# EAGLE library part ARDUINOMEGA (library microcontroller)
The Arduino Mega is a microcontroller board based on the ATmega1280. - 54 digital input/output pins (of which 14 can be used as PWM outputs) - 16 analog inputs - 4 UARTs (hardware serial ports) - 16 MHz crystal oscillator - USB connection - power jack - ICSP header - reset button It contains everything needed to support the microcontroller; simply connect it to a computer with a USB cable or power it with a AC-to-DC adapter or battery to get started. The Mega is compatible with most shields designed for the Arduino Duemilanove or Diecimila. http://arduino.cc/en/Main/ArduinoBoardMega
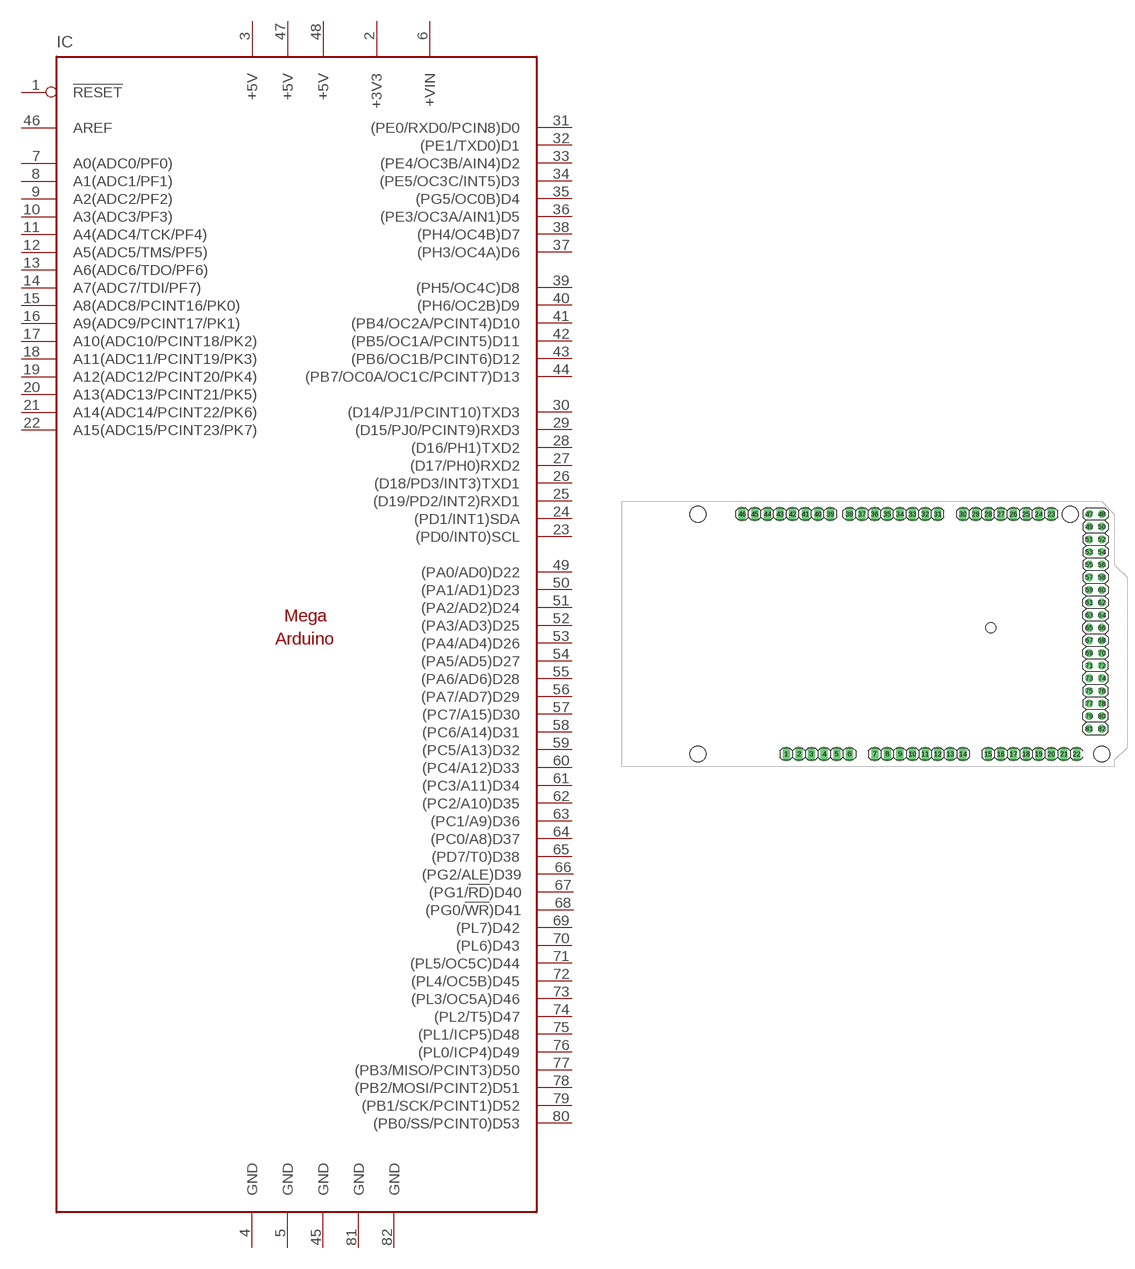
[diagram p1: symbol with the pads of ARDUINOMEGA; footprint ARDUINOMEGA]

Designator prefix IC

## ARDUINOMEGA  [ARDUINOMEGA]
1  !RESET
2  +3V3  pwr
3  +5V  pwr
4  GND  pwr
5  GND  pwr
6  +VIN  pwr
7  A0(ADC0/PF0)
8  A1(ADC1/PF1)
9  A2(ADC2/PF2)
10  A3(ADC3/PF3)
11  A4(ADC4/TCK/PF4)
12  A5(ADC5/TMS/PF5)
13  A6(ADC6/TDO/PF6)
14  A7(ADC7/TDI/PF7)
15  A8(ADC8/PCINT16/PK0)
16  A9(ADC9/PCINT17/PK1)
17  A10(ADC10/PCINT18/PK2)
18  A11(ADC11/PCINT19/PK3)
19  A12(ADC12/PCINT20/PK4)
20  A13(ADC13/PCINT21/PK5)
21  A14(ADC14/PCINT22/PK6)
22  A15(ADC15/PCINT23/PK7)
23  (PD0/INT0)SCL
24  (PD1/INT1)SDA
25  (D19/PD2/INT2)RXD1
26  (D18/PD3/INT3)TXD1
27  (D17/PH0)RXD2
28  (D16/PH1)TXD2
29  (D15/PJ0/PCINT9)RXD3
30  (D14/PJ1/PCINT10)TXD3
31  (PE0/RXD0/PCIN8)D0
32  (PE1/TXD0)D1
33  (PE4/OC3B/AIN4)D2
34  (PE5/OC3C/INT5)D3
35  (PG5/OC0B)D4
36  (PE3/OC3A/AIN1)D5
37  (PH3/OC4A)D6
38  (PH4/OC4B)D7
39  (PH5/OC4C)D8
40  (PH6/OC2B)D9
41  (PB4/OC2A/PCINT4)D10
42  (PB5/OC1A/PCINT5)D11
43  (PB6/OC1B/PCINT6)D12
44  (PB7/OC0A/OC1C/PCINT7)D13
45  GND  pwr
46  AREF
47  +5V  pwr
48  +5V  pwr
49  (PA0/AD0)D22
50  (PA1/AD1)D23
51  (PA2/AD2)D24
52  (PA3/AD3)D25
53  (PA4/AD4)D26
54  (PA5/AD5)D27
55  (PA6/AD6)D28
56  (PA7/AD7)D29
57  (PC7/A15)D30
58  (PC6/A14)D31
59  (PC5/A13)D32
60  (PC4/A12)D33
61  (PC3/A11)D34
62  (PC2/A10)D35
63  (PC1/A9)D36
64  (PC0/A8)D37
65  (PD7/T0)D38
66  (PG2/ALE)D39
67  (PG1/!RD!)D40
68  (PG0/!WR!)D41
69  (PL7)D42
70  (PL6)D43
71  (PL5/OC5C)D44
72  (PL4/OC5B)D45
73  (PL3/OC5A)D46
74  (PL2/T5)D47
75  (PL1/ICP5)D48
76  (PL0/ICP4)D49
77  (PB3/MISO/PCINT3)D50
78  (PB2/MOSI/PCINT2)D51
79  (PB1/SCK/PCINT1)D52
80  (PB0/SS/PCINT0)D53
81  GND  pwr
82  GND  pwr

## Footprint ARDUINOMEGA (pad centres in mm)
drill 1.016 long: 1 33.02,2.54; 2 35.56,2.54; 3 38.1,2.54; 4 40.64,2.54; 5 43.18,2.54; 6 45.72,2.54; 7 50.8,2.54; 8 53.34,2.54; 9 55.88,2.54; 10 58.42,2.54; 11 60.96,2.54; 12 63.5,2.54; 13 66.04,2.54; 14 68.58,2.54; 15 73.66,2.54; 16 76.2,2.54; 17 78.74,2.54; 18 81.28,2.54; 19 83.82,2.54; 20 86.36,2.54; 21 88.9,2.54; 22 91.44,2.54; 23 86.36,50.8; 24 83.82,50.8; 25 81.28,50.8; 26 78.74,50.8; 27 76.2,50.8; 28 73.66,50.8; 29 71.12,50.8; 30 68.58,50.8; 31 63.5,50.8; 32 60.96,50.8; 33 58.42,50.8; 34 55.88,50.8; 35 53.34,50.8; 36 50.8,50.8; 37 48.26,50.8; 38 45.72,50.8; 39 41.91,50.8; 40 39.37,50.8; 41 36.83,50.8; 42 34.29,50.8; 43 31.75,50.8; 44 29.21,50.8; 45 26.67,50.8; 46 24.13,50.8
drill 1.016 octagon: 47 93.98,50.8; 48 96.52,50.8; 49 93.98,48.26; 50 96.52,48.26; 51 93.98,45.72; 52 96.52,45.72; 53 93.98,43.18; 54 96.52,43.18; 55 93.98,40.64; 56 96.52,40.64; 57 93.98,38.1; 58 96.52,38.1; 59 93.98,35.56; 60 96.52,35.56; 61 93.98,33.02; 62 96.52,33.02; 63 93.98,30.48; 64 96.52,30.48; 65 93.98,27.94; 66 96.52,27.94; 67 93.98,25.4; 68 96.52,25.4; 69 93.98,22.86; 70 96.52,22.86; 71 93.98,20.32; 72 96.52,20.32; 73 93.98,17.78; 74 96.52,17.78; 75 93.98,15.24; 76 96.52,15.24; 77 93.98,12.7; 78 96.52,12.7; 79 93.98,10.16; 80 96.52,10.16; 81 93.98,7.62; 82 96.52,7.62
hole 3.2 at 15.24,50.8
hole 3.2 at 15.24,2.54
hole 3.2 at 90.17,50.8
hole 3.2 at 96.52,2.54
hole 2 at 74.168,27.94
